TYPE STR_NDI :
STRUCT
//	Heartbeat	,	
	AV101_OPEN	,	
	AV101_CLOSE	,	
	AV102_OPEN	,	
	AV102_CLOSE	,	
	AV103_OPEN	,
	AV103_CLOSE	,
	AV104_OPEN	,
	AV104_CLOSE	,
	AV105_OPEN	,
	AV105_CLOSE	,
	AV106_OPEN	,
	AV106_CLOSE	,
	CY1_OPEN	,
	CY1_CLOSE	,
	CY2_OPEN	,
	CY2_CLOSE	,
	GV1_OPEN	,
	GV1_CLOSE	,
	Lid_Closed	,
	Water_Leak_Sensor01	,
	Water_Leak_Sensor02	,
	Water_Leak_Sensor03	,
	Water_Leak_Sensor04	,
//	WAFER_CHECK_SENSOR1	,
//	WAFER_CHECK_SENSOR2	,
//	WAFER_CHECK_SENSOR3	,
//	WAFER_CHECK_SENSOR4	,
//	PS10_H_ALM	,	
//	PS10_L_ALM	,
//	PS11_H_ALM	,
//	PS11_L_ALM	,
//	PS12_H_ALM		,
//	PS12_L_ALM	,
//	LID_heater_OT	,
//	Chamber_heater_OT	,
	Chiller_Controller_ALM	,
	PG_PS1_Pressure_Switch_Up_Limit	,
	PG_PS1_Pressure_Switch_Down_Limit	,
	PG_PS2_Pressure_Switch_Up_Limit	,
	PG_PS2_Pressure_Switch_Down_Limit	,
	PG_PS3_Pressure_Switch_Up_Limit	,
	PG_PS3_Pressure_Switch_Down_Limit	,
	PG_PS4_Pressure_Switch_Up_Limit	,
	PG_PS4_Pressure_Switch_Down_Limit	,
	PG_PS5_Pressure_Switch_Up_Limit	,
	PG_PS5_Pressure_Switch_Down_Limit	,
	PG_PS6_Pressure_Switch_Up_Limit	,
	PG_PS6_Pressure_Switch_Down_Limit	,
	PG_PS7_Pressure_Switch_Up_Limit	,
	PG_PS7_Pressure_Switch_Down_Limit	,
	PG_PS8_Pressure_Switch_Up_Limit	,
	PG_PS8_Pressure_Switch_Down_Limit	,
	PG_PS9_Pressure_Switch_Up_Limit	,
	PG_PS9_Pressure_Switch_Down_Limit	,
	MS1_ALM	,
	PS1_Pressure_Switch	,
	PS2_Pressure_Switch	,
(*	Forline_Heater1_OT	,
	Forline_Heater2_OT	,
	Forline_Heater3_OT	,
	Forline_Heater4_OT	,
	Forline_Heater5_OT	,
	Forline_Heater6_OT	,
	Forline_Heater7_OT	,
	Forline_Heater8_OT	,
	Turbo_Pump_Heater_OT	,
	Pendulum_Valve_Heater_OT	,
	IGS_Heater_OT	,
	Tape_Heater_OT	,
//	Foreline_Heater_OT	,
	Gate_Valve_OT	,
	Stage_Heater_OT	,
*)	CDA_OK	,
	Lift_Pin_Middle1	,
	Lift_Pin_Middle2	,
//	FL01B2	,
//	FL01B4	,
	FL02B2	,
//	FL02B4	,
	FL03B2	,
//	FL03B4	,
	FL04B2	,
//	FL04B4	,
//	DP01_OUTPUT1	,
//	DP01_OUTPUT2	,
//	MaualEndStepFeedBack	,
	AV1		,
	AV2		,
	AV3		,
	AV4		,
	AV6		,
	AV7		,
	AV9		,
	AV10	,
	AV11	,
	AV12	,
	AV13	,
	AV14	,
	AV16	,
	AV17	,
	AV19	,
	AV20	,
	AV22	,
	AV23	,
	AV25	,
	AV26	,
	AV27	,
	AV5		,
	AV8		,
	AV15	,
	AV18	,
	AV21	,
	AV24	,
	GD1_ALM	,
	GD2_ALM	,
	GD_FAULT,
	Robot_Extend_TO_PM,
	SYS_CDA_OK,
	SYS_N2_OK,
	TM_Lid_Closed:BOOL;
END_STRUCT
END_TYPE
